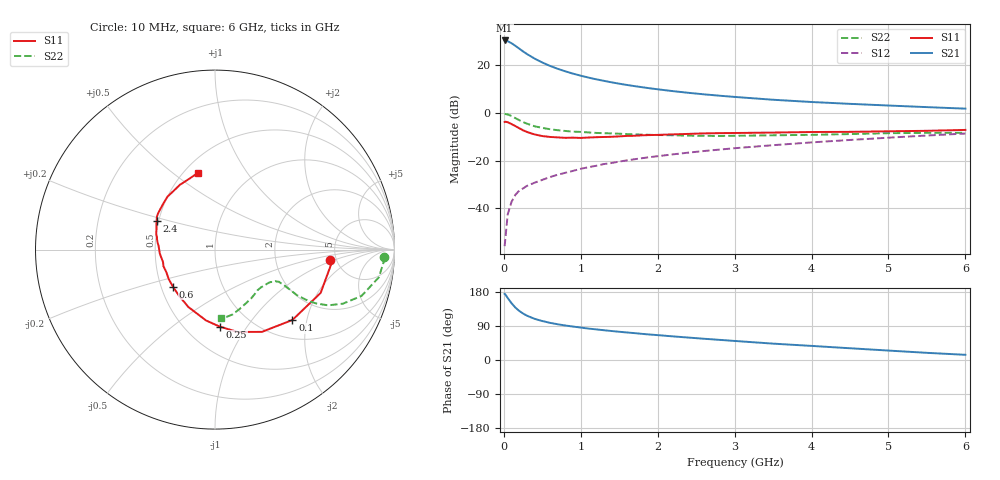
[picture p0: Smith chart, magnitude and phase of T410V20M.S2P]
! Infineon Technologies  Discrete & RF Semiconductors
! BFR182T
! Si NPN RF Bipolar Junction Transistor in SC75
! VCE = 10 V  IC = 20 mA
! Common Emitter S-Parameters:  October  1999
# GHz  S  MA  R  50
!  f  S11  S21  S12  S22
! GHz  MAG  ANG  MAG  ANG  MAG  ANG  MAG  ANG
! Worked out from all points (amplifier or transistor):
!   36 points, 10 MHz to 6 GHz, reference 50 ohm
!   highest |S21| = 30.4 dB at 10 MHz (marker M1)
!   |S21| within 3 dB of that: start of sweep to 181.8 MHz
!   unconditionally stable (mu >= 1): 791.5 MHz to 3.93 GHz
!   at 250 MHz: K = 0.59, MSG = 28.7 dB, |S12| = -31.7 dB
!   at 1.4 GHz: K = 1.08, MAG = 15.2 dB, |S12| = -21.0 dB
!   at 6 GHz: K = 0.87, MSG = 5.2 dB, |S12| = -8.7 dB
!   S11 on the Smith chart (normalised r, x): 10 MHz: 4.43, -0.90; 100 MHz: 1.38, -1.64; 250 MHz: 0.72, -0.76; 600 MHz: 0.58, -0.26; 2.4 GHz: 0.49, +0.18; 6 GHz: 0.59, +0.62
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0.01  0.6444 -5.3  32.96 174.6  0.0016 61.5  0.9433 -2.5
0.02  0.6513 -7.6  32.59 172.9  0.0023 83.1  0.9442 -3.7
0.05  0.6362 -22.3  31.74 163.6  0.0074 79.9  0.9259 -9.6
0.1  0.5828 -42.3  28.84 149.9  0.0136 73.2  0.8567 -17.5
0.15  0.5277 -60.3  25.4 138.3  0.0191 66.9  0.7741 -22.9
0.2  0.476 -74.6  22.23 129.5  0.0234 66.6  0.7035 -26.2
0.25  0.4302 -86.4  19.43 122.6  0.026 63.3  0.6401 -28.0
0.3  0.3978 -97.3  17.14 117.0  0.0294 63.3  0.5938 -28.8
0.4  0.3524 -114.9  13.73 108.6  0.0343 62.7  0.5233 -29.1
0.5  0.3259 -128.0  11.37 102.8  0.0393 65.0  0.4828 -28.3
0.6  0.3122 -138.8  9.646 98.1  0.0451 65.3  0.4538 -27.8
0.8  0.299 -155.2  7.42 91.0  0.0554 67.2  0.4168 -27.0
0.9  0.3017 -162.0  6.631 88.2  0.0607 68.1  0.4038 -26.9
1.1  0.3037 -172.5  5.493 82.9  0.0724 68.6  0.3884 -27.3
1.3  0.3117 179.3  4.693 78.6  0.0843 69.0  0.3745 -28.3
1.6  0.3281 169.9  3.845 72.6  0.1008 68.7  0.3584 -30.3
2.2  0.3536 157.4  2.851 62.3  0.1348 68.1  0.3387 -36.5
2.4  0.3618 154.0  2.631 59.2  0.1465 67.4  0.3322 -39.0
3.5  0.3858 138.1  1.882 43.2  0.2098 63.0  0.3381 -53.3
4.5  0.3995 125.9  1.544 31.0  0.27 58.0  0.359 -68.0
5.5  0.42 109.9  1.318 18.9  0.3346 52.5  0.3801 -80.0
6  0.4387 102.3  1.225 13.7  0.3685 49.0  0.3811 -84.7
